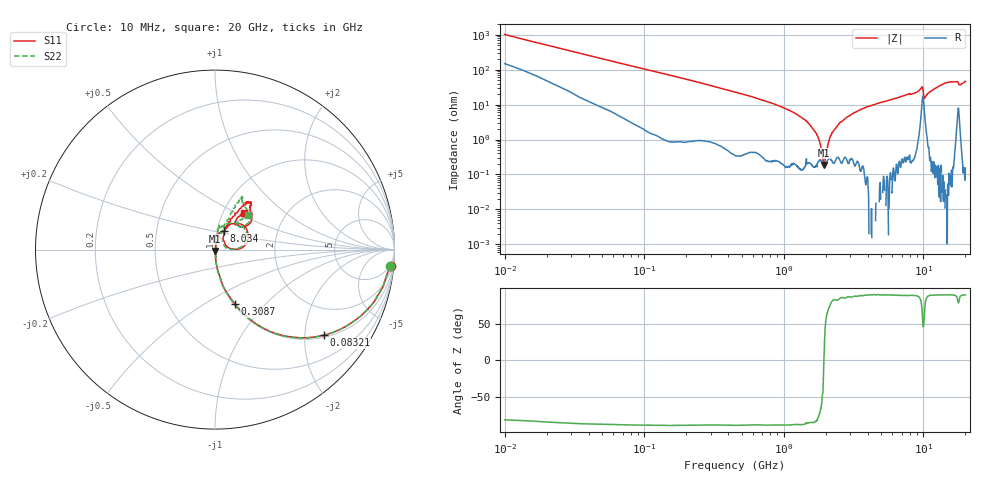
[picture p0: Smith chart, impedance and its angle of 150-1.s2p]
!Keysight Technologies,P5008B,MY61100088,A.16.20.02
!Date: Monday, May 27, 2024 17:17:32
!Correction: S11(C* 2-Port  )
!S21(C* 2-Port  )
!S12(C* 2-Port  )
!S22(C* 2-Port  )
!S2P File: Measurements: S11, S21, S12, S22:Log Frequency Sweep
# Hz S  dB  R 50
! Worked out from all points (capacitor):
!   1601 points, 10 MHz to 20 GHz, reference 50 ohm
!   read as one part in series: C = 15.8 pF near 10.39 MHz
!   lowest |Z| = 188 mohm at 1.95 GHz (marker M1)
!   series resonance near 1.938 GHz, so ESL is about 430 pH
!   S11 on the Smith chart (normalised r, x): 10 MHz: 4, -20; 83.21 MHz: 1.06, -2.50; 308.7 MHz: 1.02, -0.68; 8.034 GHz: 1.08, +0.23; 20 GHz: 1.25, +0.55
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1e7  -0.15 -5.5  -20.33 76.1  -20.34 76.2  -0.17 -5.5
3.555162e7  -0.64 -18.9  -9.76 68.0  -9.77 68.0  -0.65 -19.0
8.320743e7  -2.25 -38.1  -4.18 50.5  -4.19 50.5  -2.25 -38.2
1.263918e8  -3.92 -49.7  -2.37 39.5  -2.38 39.5  -3.91 -49.7
3.087378e8  -9.86 -70.0  -0.53 18.5  -0.54 18.5  -9.87 -70.2
4.472136e8  -12.99 -76.5  -0.26 12.7  -0.26 12.7  -12.98 -76.7
1.108091e9  -22.89 -85.2  -0.03 3.6  -0.04 3.6  -22.87 -84.7
1.589917e9  -31.04 -86.5  -0.01 0.9  -0.02 0.9  -30.61 -81.0
1.950247e9  -41.97 -84.3  -0.00 -0.5  -0.01 -0.5  -39.41 -62.0
2.114282e9  -49.78 4.3  -0.00 -1.1  -0.01 -1.1  -42.66 -10.9
2.25968e9  -43.06 76.5  0.00 -1.6  -0.01 -1.6  -41.92 39.8
2.496738e9  -34.95 76.9  0.00 -2.3  -0.01 -2.3  -35.04 64.2
2.824976e9  -30.82 81.7  -0.00 -3.3  -0.01 -3.3  -30.44 72.5
3.846973e9  -25.05 90.7  -0.00 -6.1  -0.02 -6.1  -24.03 74.8
5.652411e9  -21.00 78.8  -0.02 -10.1  -0.03 -10.1  -21.01 79.5
8.03353e9  -18.66 64.2  -0.03 -15.5  -0.04 -15.5  -18.60 78.6
9.622897e9  -14.51 50.4  -0.53 -22.1  -0.54 -22.2  -14.63 55.2
1.048196e10  -22.81 52.0  -0.13 -16.7  -0.14 -16.8  -23.48 63.0
1.427404e10  -10.37 55.6  -0.33 -28.7  -0.34 -28.7  -10.36 64.6
1.685609e10  -10.26 50.4  -0.39 -33.0  -0.40 -33.1  -10.34 59.8
1.853616e10  -14.61 52.7  -0.17 -33.7  -0.18 -33.8  -14.41 51.4
2e10  -11.69 51.9  -0.25 -39.4  -0.26 -39.5  -11.50 46.7
